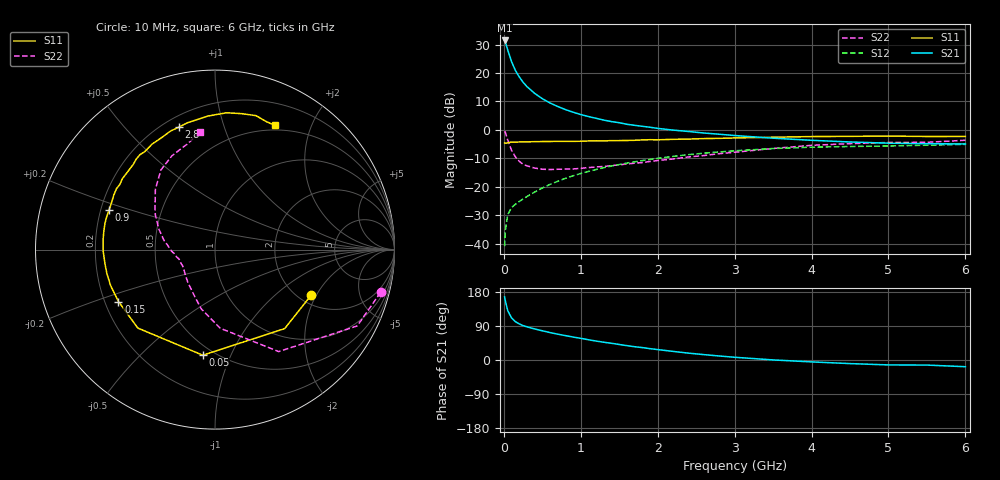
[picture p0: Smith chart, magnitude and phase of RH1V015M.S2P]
! SIEMENS Small Signal Semiconductors
! BFR106
! Si NPN RF Bipolar Junction Transistor in SOT23
! VCE = 1 V  IC = 15 mA
! Common Emitter S-Parameters:  August  1996
# GHz  S  MA  R  50
!  f  S11  S21  S12  S22
! GHz  MAG  ANG  MAG  ANG  MAG  ANG  MAG  ANG
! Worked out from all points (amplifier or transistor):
!   36 points, 10 MHz to 6 GHz, reference 50 ohm
!   highest |S21| = 31.4 dB at 10 MHz (marker M1)
!   |S21| within 3 dB of that: start of sweep to 46.71 MHz
!   unconditionally stable (mu >= 1): 380.7 MHz to 3.176 GHz; 4.042 GHz to end of sweep
!   at 250 MHz: K = 0.85, MSG = 20.5 dB, |S12| = -24.3 dB
!   at 1.4 GHz: K = 1.10, MAG = 5.8 dB, |S12| = -12.7 dB
!   at 6 GHz: K = 1.03, MAG = -0.9 dB, |S12| = -5.1 dB
!   S11 on the Smith chart (normalised r, x): 10 MHz: 2.31, -1.81; 50 MHz: 0.44, -0.79; 150 MHz: 0.26, -0.24; 900 MHz: 0.23, +0.17; 2.8 GHz: 0.26, +0.72; 6 GHz: 0.44, +1.50
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0.01  0.5928 -25.4  37.29 166.5  0.0091 79.7  0.9528 -14.5
0.02  0.5869 -48.6  34.85 155.3  0.0173 69.6  0.8995 -28.2
0.05  0.5923 -96.6  25.52 130.5  0.0323 53.0  0.67 -58.0
0.1  0.6132 -134.5  15.89 111.1  0.0435 44.5  0.4393 -86.2
0.15  0.6107 -151.7  11.12 101.2  0.0496 44.6  0.3378 -103.3
0.2  0.6151 -161.0  8.571 95.3  0.0554 46.8  0.2811 -114.2
0.25  0.6169 -167.3  6.886 90.8  0.0613 49.3  0.2495 -124.1
0.3  0.6178 -172.0  5.78 87.5  0.0677 51.8  0.2345 -130.7
0.4  0.623 -179.2  4.396 82.0  0.081 55.5  0.2141 -141.5
0.5  0.6259 175.3  3.541 77.1  0.0955 57.4  0.2042 -148.8
0.6  0.6278 170.6  2.976 72.4  0.1105 58.5  0.2019 -153.4
0.7  0.6302 166.4  2.584 68.1  0.1254 59.2  0.204 -157.5
0.9  0.63 159.3  2.051 60.6  0.1567 58.9  0.2064 -164.9
1.1  0.6403 151.9  1.718 53.4  0.1871 57.5  0.2187 -169.5
1.3  0.6425 145.5  1.488 46.8  0.2174 55.3  0.2287 -174.7
1.6  0.6533 136.8  1.258 37.9  0.2616 51.6  0.2524 178.7
2.2  0.6846 120.7  0.994 22.7  0.3435 42.4  0.309 164.6
2.8  0.7117 106.3  0.841 10.6  0.411 32.6  0.3833 150.0
3.5  0.7452 93.0  0.717 0.2  0.4714 21.4  0.4729 134.6
4.5  0.7721 78.7  0.615 -9.5  0.5122 6.8  0.5749 114.7
5.5  0.768 67.9  0.574 -13.4  0.5397 -2.1  0.6068 104.9
6  0.7692 64.1  0.568 -17.7  0.5577 -8.6  0.6597 97.1
